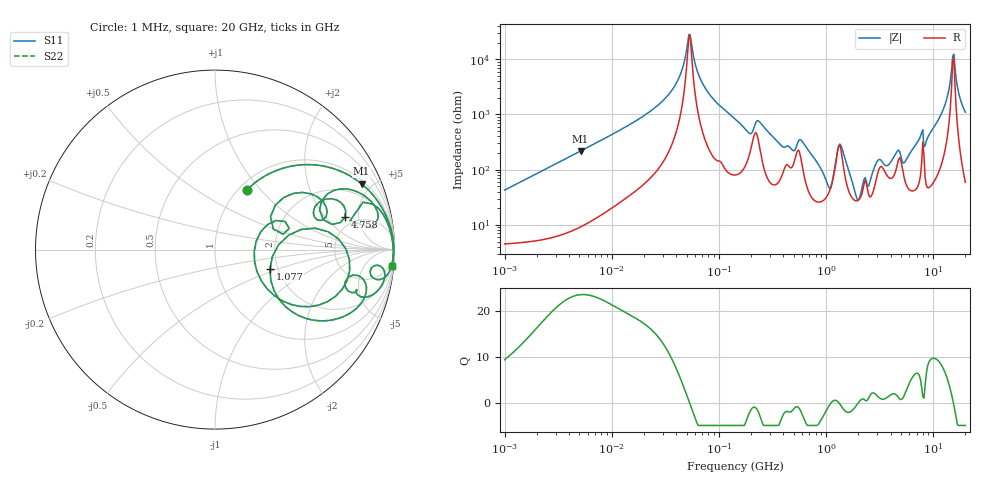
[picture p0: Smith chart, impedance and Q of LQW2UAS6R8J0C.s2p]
!Murata Part Number: LQW2UAS6R8J0C
!These Parameters are Measured in Series Mode Connection
!  o--[Z]--o
!Port1  Port2
!  o-------o
!Freq. Start=1[MHz] Stop=20[GHz], 401[Steps]
# Hz S RI R 50
!Freq.(Hz) S11(Real) S11(Imag) S21(Real) S21(Imag) S12(Real) S12(Imag) S22(Real) S22(Imag)
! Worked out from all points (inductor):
!   401 points, 1 MHz to 20 GHz, reference 50 ohm
!   read as one part in series: L = 6.76 uH near 1.051 MHz
!   highest Q = 23.7 at 5.125 MHz (marker M1), where L = 6.77 uH
!   self-resonance near 52.53 MHz
!   S11 on the Smith chart (normalised r, x): 1 MHz: 1.09, +0.85; 1.077 GHz: 1.81, -0.44; 4.758 GHz: 4.07, +3.32; 20 GHz: 2, -22
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1000000  0.1795 0.3343  0.8205 -0.3343  0.8205 -0.3343  0.1795 0.3343
5124718  0.8163 0.3667  0.1837 -0.3667  0.1837 -0.3667  0.8163 0.3667
5253183  0.8233 0.3609  0.1767 -0.3609  0.1767 -0.3609  0.8233 0.3609
2.759593e7  0.9912 0.0644  0.00877 -0.0644  0.00877 -0.0644  0.9912 0.0644
4.100967e7  0.9958 0.0245  0.00416 -0.0245  0.00416 -0.0245  0.9958 0.0245
5.384738e7  0.9966 -0.00115  0.00335 0.00115  0.00335 0.00115  0.9966 -0.00115
7.247621e7  0.9954 -0.0299  0.00459 0.0299  0.00459 0.0299  0.9954 -0.0299
1.414214e8  0.9748 -0.1155  0.0252 0.1155  0.0252 0.1155  0.9748 -0.1155
7.429123e8  0.7331 -0.3651  0.2669 0.3651  0.2669 0.3651  0.7331 -0.3651
1.077026e9  0.3062 -0.1079  0.6938 0.1079  0.6938 0.1079  0.3062 -0.1079
1.218959e9  0.5584 0.1191  0.4416 -0.1191  0.4416 -0.1191  0.5584 0.1191
1.345858e9  0.7491 -0.057  0.2509 0.057  0.2509 0.057  0.7491 -0.057
1.640665e9  0.4758 -0.3167  0.5242 0.3167  0.5242 0.3167  0.4758 -0.3167
2.000048e9  0.2187 -0.00947  0.7813 0.00947  0.7813 0.00947  0.2187 -0.00947
2.691977e9  0.4358 0.3127  0.5642 -0.3127  0.5642 -0.3127  0.4358 0.3127
3.902654e9  0.5778 0.2627  0.4222 -0.2627  0.4222 -0.2627  0.5778 0.2627
4.75752e9  0.724 0.1807  0.276 -0.1807  0.276 -0.1807  0.724 0.1807
5.519454e9  0.6263 0.3102  0.3737 -0.3102  0.3737 -0.3102  0.6263 0.3102
8.834765e9  0.9067 0.2335  0.0933 -0.2335  0.0933 -0.2335  0.9067 0.2335
1.280807e10  0.9855 0.0669  0.0145 -0.0669  0.0145 -0.0669  0.9855 0.0669
1.523182e10  0.9927 0.00476  0.0073 -0.00476  0.0073 -0.00476  0.9927 0.00476
2e10  0.9871 -0.0893  0.0129 0.0893  0.0129 0.0893  0.9871 -0.0893
